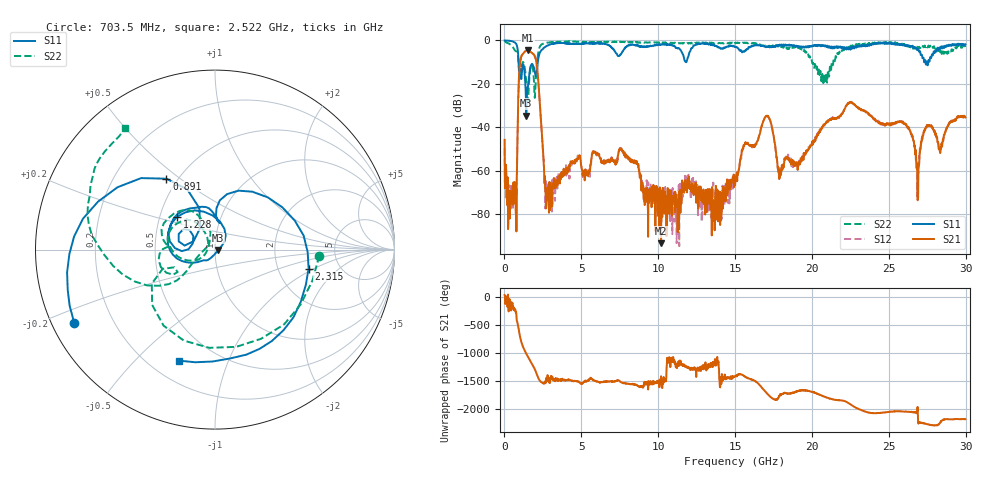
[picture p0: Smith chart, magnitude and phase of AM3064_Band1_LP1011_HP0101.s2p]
# Hz S DB R 50.0
!freq dBS11 angS11 dBS21 angS21 dBS12 angS12 dBS22 angS22
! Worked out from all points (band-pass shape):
!   1600 points, 10 MHz to 29.98 GHz, reference 50 ohm
!   highest |S21| = -4.59 dB at 1.51 GHz (marker M1); lowest = -93.5 dB at 10.19 GHz (marker M2)
!   |S21| within 3 dB of the highest: 1.089 GHz to 1.988 GHz (898.7 MHz wide, 58.4 % of centre)
!   lowest |S11| = -34.6 dB at 1.416 GHz (marker M3), VSWR 1.04, Z = 51.9 - j0.236 ohm
!   |S11| at or under -10 dB: 916.9 MHz to 2.165 GHz (1.248 GHz wide, 81 % of centre); 27.39288 GHz to 27.46049 GHz (67.61 MHz wide, 0.247 % of centre); 27.49058 GHz to 27.56429 GHz (73.71 MHz wide, 0.268 % of centre)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
!   |S22| runs from -27.9 to -0.4 dB; largest |S21 - S12| = 0.0079
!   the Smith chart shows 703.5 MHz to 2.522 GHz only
!   S11 on the Smith chart (normalised r, x): 703.5 MHz: 0.07, -0.24; 891 MHz: 0.44, +0.45; 1.228 GHz: 0.61, +0.24; 2.315 GHz: 2.99, -0.88; 2.522 GHz: 0.32, -0.68
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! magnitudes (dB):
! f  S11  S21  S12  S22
! 10 MHz  0.0  -45.8  -49.7  -0.4
! 703.5 MHz  -1.1  -71.6  -67.1  -4.7
! 891 MHz  -6.4  -29.8  -29.7  -8.0
! 1.228 GHz  -11.1  -6.0  -5.9  -10.1
! 1.416 GHz  -34.6  -4.7  -4.7  -18.9
! 1.51 GHz  -21.8  -4.6  -4.6  -26.1
! 2.315 GHz  -5.5  -30.7  -30.5  -2.7
! 2.522 GHz  -3.7  -52.2  -53.4  -1.5
! 2.822 GHz  -2.3  -72.0  -68.2  -1.0
! 5.015 GHz  -1.4  -58.2  -59.0  -0.8
! 7.601 GHz  -6.1  -49.7  -49.7  -0.7
! 10 GHz  -2.0  -80.8  -68.6  -0.9
! 10.19 GHz  -2.0  -93.5  -71.8  -1.0
! 15 GHz  -2.9  -66.7  -63.8  -1.4
! 17.03 GHz  -3.1  -34.8  -34.8  -2.9
! 17.93 GHz  -2.0  -60.9  -58.8  -2.3
! 19.99 GHz  -2.9  -47.5  -47.5  -9.4
! 22.45 GHz  -3.2  -28.7  -28.4  -3.5
! 25 GHz  -1.1  -38.3  -38.4  -1.1
! 26.87 GHz  -4.3  -73.5  -63.1  -3.1
! 27.47 GHz  -9.7  -39.9  -39.0  -2.5
! 29.98 GHz  -1.8  -35.5  -35.1  -3.1
